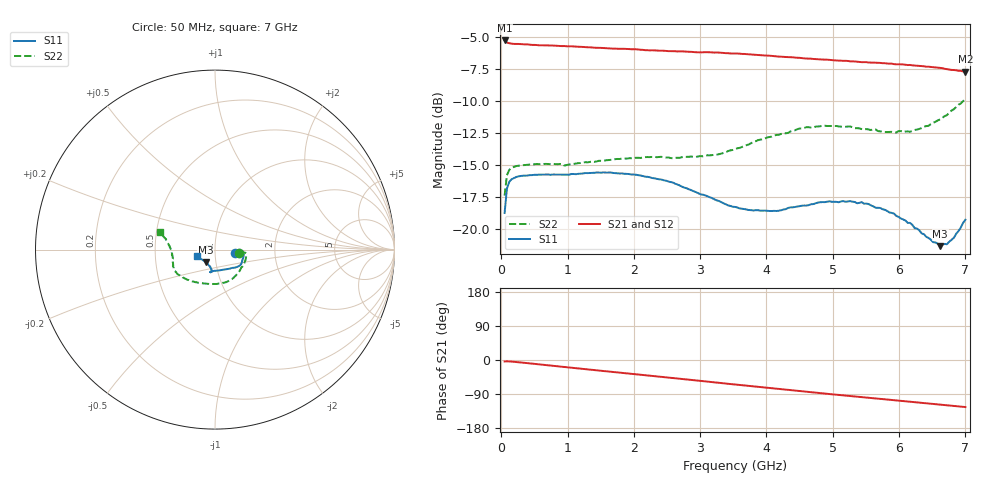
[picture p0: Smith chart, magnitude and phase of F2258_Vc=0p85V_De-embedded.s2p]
! Integrated Device Technology
! Corporate Headquarters
! 6024 Silver Creek Valley Road
! San Jose, CA 95138  USA
! Phone:  1-408-284-8200
! Toll Free:  1-800-223-1366
! Webpage:  http://www.idt.com/
! Timing and RF Division
! 515 Groton Road, Suite 102
! Westford, MA 01886-6024
! Device:  F2258
! Description: Voltage Variable RF Attenuator
! Frequency:  50.0 -  6000.00 MHz
! Package:  3x3 mm Thin QFN Plastic Package: 16 pin
! Ports:  2 RF, 2 DC
!  Pin  1  = NC
!  Pin  2  = NC
!  Pin  3  = RF2  = Port 2
!  Pin  4  = GND
!  Pin  5  = Vdd
!  Pin  6  = NC
!  Pin  7  = VCTRL
!  Pin  8  = NC
!  Pin  9  = GND
!  Pin 10  = RF1  = Port 1
!  Pin 11  = NC
!  Pin 12  = NC
!  Pin 13  = NC
!  Pin 14  = NC
!  Pin 15  = NC
!  Pin 16  = NC
! Vcntrl:  0.850 Volts
! Vdd:  +3.300 Volts
! Current:  1.139 mA
! Data:  The device was measured on a the F2258 evaluation board which has
!  individual transmission lines to the RF pins.  Data was collected
!  using a calibrated network analyzer.  The evaluation board was
!  de-embedded using a TRL calibration technique.
!  The reference plane is the edge of the package pin.
! Misc:  SN 10
!  Action Tracker AT0285
! Date Measured:  2014-12-10
! Date:  2016-01-13  MJV
! Note:
!  Integrated Device Technology supplies this data as a sample of measured
!  data at the package pin for this product.  Your particular data for this
!  product may vary.
!  Data was taken at 25 degrees C.
!  Integrated Device Technology reserves the right to change this data at anytime.
!Freq_(GHz)  S11M_(dB)  S11P_(deg)  S21M_(dB)  S21P_(deg)  S12M_(dB)  S12P_(deg)  S22M_(dB)  S22P_(deg)
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# GHz S dB R 50
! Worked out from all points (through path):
!   201 points, 50 MHz to 7 GHz, reference 50 ohm
!   highest |S21| = -5.23 dB at 50 MHz (marker M1); lowest = -7.7 dB at 7 GHz (marker M2)
!   group delay of S21, straight-line fit = 49 ps
!   lowest |S11| = -21.3 dB at 6.618 GHz (marker M3), VSWR 1.19, Z = 44.8 - j6.24 ohm
!   |S11| at or under -10 dB: start of sweep to end of sweep
!   |S22| runs from -17.4 to -9.8 dB; largest |S21 - S12| = 0.0032
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0.05  -18.75 -9.7  -5.23 -3.8  -5.26 -3.9  -17.38 -8.1
0.08475  -16.84 -5.5  -5.40 -3.5  -5.41 -3.5  -15.79 -5.7
0.1195  -16.31 -4.5  -5.45 -3.7  -5.47 -3.8  -15.37 -6.0
0.189  -16.02 -5.1  -5.50 -4.7  -5.53 -4.7  -15.14 -7.8
0.6755  -15.73 -14.1  -5.62 -13.4  -5.63 -13.4  -14.90 -23.6
0.9535  -15.75 -20.5  -5.67 -18.5  -5.68 -18.5  -15.04 -33.6
1.2315  -15.66 -24.7  -5.74 -23.5  -5.75 -23.5  -14.80 -42.4
1.6485  -15.57 -30.0  -5.86 -31.0  -5.86 -31.0  -14.58 -54.2
2.37825  -16.10 -37.7  -6.04 -43.8  -6.02 -43.8  -14.36 -74.0
3.0385  -17.31 -50.2  -6.16 -55.7  -6.17 -55.7  -14.31 -96.2
3.525  -18.27 -66.4  -6.25 -64.7  -6.28 -64.7  -13.76 -115.5
4.1505  -18.59 -89.5  -6.49 -76.0  -6.52 -76.0  -12.63 -136.5
4.7065  -18.05 -100.1  -6.68 -85.7  -6.71 -85.7  -12.04 -149.5
5.2625  -17.82 -101.3  -6.87 -95.1  -6.90 -95.0  -11.97 -158.6
5.43625  -17.90 -99.8  -6.93 -97.9  -6.94 -97.9  -12.17 -161.5
5.85325  -18.70 -99.1  -7.05 -104.9  -7.06 -104.9  -12.40 -170.0
6.166  -19.52 -102.5  -7.15 -110.2  -7.17 -110.2  -12.39 -177.2
6.2355  -19.94 -104.2  -7.20 -111.3  -7.20 -111.4  -12.24 -179.2
6.61775  -21.34 -126.2  -7.38 -117.9  -7.40 -117.9  -11.42 170.7
6.722  -21.19 -134.8  -7.48 -119.7  -7.46 -119.7  -11.08 167.9
6.82625  -20.68 -144.5  -7.55 -121.4  -7.52 -121.4  -10.62 166.0
7  -19.27 -160.1  -7.68 -124.2  -7.66 -124.2  -9.80 162.3
